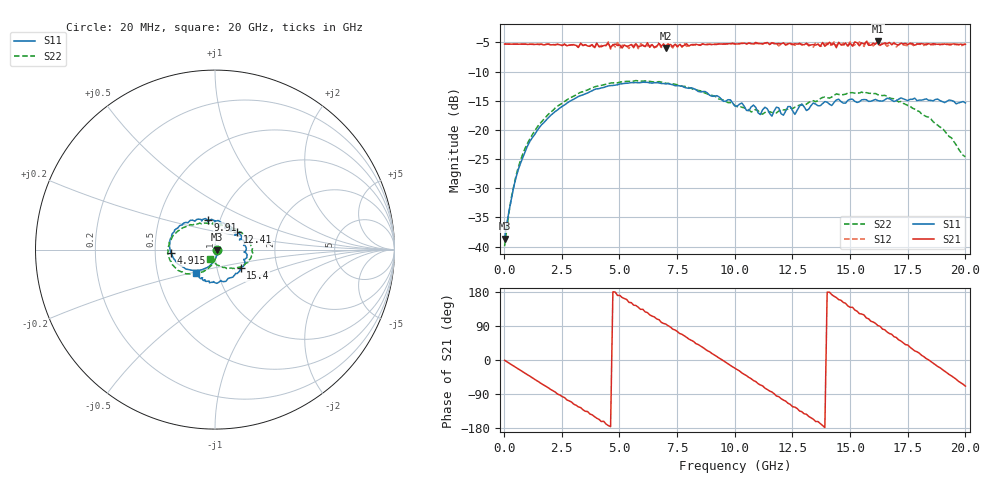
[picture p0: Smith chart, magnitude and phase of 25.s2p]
!Agilent Technologies,N5230A,US43500223,A.07.50.48
!Agilent N5230A: A.07.50.48
!Date: Sunday, September 13, 2015 17:33:46
!Correction: S11(Full 2 Port(1,2))
!S21(Full 2 Port(1,2))
!S12(Full 2 Port(1,2))
!S22(Full 2 Port(1,2))
!S2P File: Measurements: S11, S21, S12, S22:
# Hz S  dB  R 50
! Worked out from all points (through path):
!   201 points, 20 MHz to 20 GHz, reference 50 ohm
!   highest |S21| = -4.80 dB at 16.2 GHz (marker M1); lowest = -6.0 dB at 7.013 GHz (marker M2)
!   group delay of S21, straight-line fit = 109 ps
!   lowest |S11| = -38.7 dB at 20 MHz (marker M3), VSWR 1.02, Z = 51.2 - j0.101 ohm
!   |S11| at or under -10 dB: start of sweep to end of sweep
!   |S22| runs from -39.9 to -11.5 dB; largest |S21 - S12| = 0.057
!   S11 on the Smith chart (normalised r, x): 20 MHz: 1.02, -0.00; 4.915 GHz: 0.61, -0.02; 9.91 GHz: 0.88, +0.30; 12.41 GHz: 1.25, +0.26; 15.4 GHz: 1.30, -0.27; 20 GHz: 0.78, -0.21
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2e7  -38.65 -4.8  -5.28 -0.8  -5.27 -0.8  -39.94 -4.7
5.195e8  -28.09 -79.1  -5.29 -20.0  -5.29 -20.1  -27.79 -82.3
1.019e9  -22.71 -98.7  -5.34 -39.2  -5.34 -39.2  -22.25 -98.3
2.3177e9  -16.56 -129.3  -5.31 -90.0  -5.32 -90.0  -15.93 -124.4
3.4166e9  -13.99 -149.9  -5.51 -131.2  -5.53 -133.3  -13.45 -141.9
4.9151e9  -12.26 -175.5  -5.52 170.3  -5.02 168.4  -11.94 -164.8
6.7133e9  -11.92 158.8  -5.10 106.3  -5.20 106.3  -11.72 171.0
7.013e9  -12.11 155.9  -5.98 94.5  -5.57 93.7  -12.01 167.3
7.9121e9  -12.80 143.4  -5.22 59.8  -5.67 59.0  -12.63 154.9
8.6114e9  -13.43 133.5  -5.23 33.3  -5.27 32.7  -13.50 144.0
9.9101e9  -15.40 103.8  -5.13 -18.2  -5.18 -18.1  -15.46 119.1
1.001e10  -15.92 102.8  -5.24 -21.9  -5.29 -22.4  -15.84 117.7
1.13087e10  -16.11 73.3  -5.11 -74.3  -5.08 -74.8  -17.01 81.7
1.24076e10  -16.00 39.1  -5.17 -117.2  -5.44 -116.3  -16.24 53.8
1.34066e10  -15.38 15.5  -5.37 -156.3  -5.80 -155.2  -14.99 30.9
1.43057e10  -15.28 -6.0  -5.18 168.2  -4.92 169.6  -14.07 13.7
1.54046e10  -15.16 -35.4  -5.58 122.3  -4.91 121.7  -13.66 -3.3
1.62038e10  -14.97 -61.7  -4.80 90.8  -5.29 89.5  -13.97 -15.8
1.67033e10  -14.66 -75.0  -5.00 69.9  -5.40 71.1  -14.53 -23.9
1.83017e10  -14.68 -106.1  -5.42 3.8  -5.18 3.7  -17.70 -53.3
1.91009e10  -15.32 -113.7  -5.26 -29.5  -5.34 -29.8  -20.19 -70.6
2e10  -15.37 -128.7  -5.32 -69.0  -5.24 -69.2  -24.61 -117.1
